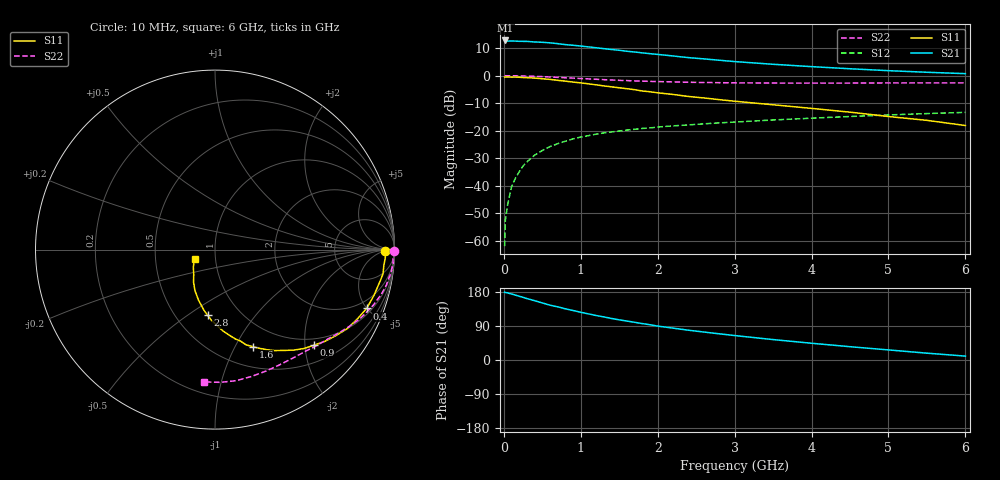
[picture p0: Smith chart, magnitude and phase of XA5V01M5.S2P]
! SIEMENS Discrete & RF Semiconductors
! BFY180
! Si NPN RF Bipolar Junction Transistor in MICRO-X
! VCE = 5 V  IC = 1.5 mA
! Common Emitter S-Parameters:  May  1997
# GHz  S  MA  R  50
!  f  S11  S21  S12  S22
! GHz  MAG  ANG  MAG  ANG  MAG  ANG  MAG  ANG
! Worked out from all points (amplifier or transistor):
!   36 points, 10 MHz to 6 GHz, reference 50 ohm
!   highest |S21| = 12.8 dB at 20 MHz (marker M1)
!   |S21| within 3 dB of that: start of sweep to 1.308 GHz
!   unconditionally stable (mu >= 1): 3.398 GHz to end of sweep
!   at 250 MHz: K = 0.10, MSG = 22.6 dB, |S12| = -32.8 dB
!   at 1.4 GHz: K = 0.58, MSG = 15.0 dB, |S12| = -20.4 dB
!   at 6 GHz: K = 1.06, MAG = 5.5 dB, |S12| = -13.3 dB
!   S11 on the Smith chart (normalised r, x): 10 MHz: 35, -4; 400 MHz: 1.36, -4.99; 900 MHz: 0.85, -2.20; 1.6 GHz: 0.72, -1.18; 2.8 GHz: 0.71, -0.60; 6 GHz: 0.79, -0.08
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0.01  0.9451 -0.4  4.292 179.0  0.0008 78.9  0.9969 -0.3
0.02  0.9477 -1.4  4.372 178.2  0.0024 87.1  0.9999 -0.6
0.05  0.9501 -2.7  4.251 177.0  0.0046 88.2  0.9971 -1.5
0.1  0.9448 -5.4  4.285 174.2  0.0096 87.2  0.9925 -3.0
0.15  0.9457 -8.2  4.252 171.3  0.0137 85.4  0.9958 -4.5
0.25  0.9275 -13.6  4.21 165.4  0.0229 81.2  0.9896 -7.5
0.3  0.9212 -16.2  4.209 162.1  0.0272 79.3  0.983 -8.9
0.4  0.9062 -21.2  4.101 156.5  0.036 76.0  0.9746 -11.7
0.5  0.8806 -26.3  4.05 150.6  0.0438 72.7  0.9626 -14.4
0.6  0.8575 -31.0  3.956 144.7  0.0515 69.7  0.9481 -16.9
0.9  0.7667 -44.0  3.574 130.6  0.0712 61.1  0.9047 -23.9
1.1  0.7122 -51.8  3.338 121.7  0.0815 56.9  0.8752 -27.9
1.4  0.6282 -62.6  2.998 109.6  0.0951 51.4  0.8364 -33.3
1.6  0.5806 -68.7  2.782 102.8  0.1029 48.5  0.8155 -36.4
2  0.4892 -79.8  2.44 89.5  0.1168 43.6  0.7831 -42.2
2.2  0.4569 -84.2  2.284 84.1  0.1227 41.3  0.772 -45.0
2.4  0.4198 -89.0  2.131 78.6  0.1278 39.6  0.7605 -47.6
2.8  0.3675 -96.5  1.911 69.1  0.1392 36.5  0.7474 -52.6
3.5  0.2966 -108.0  1.614 53.9  0.157 31.2  0.7358 -61.2
4.5  0.2177 -123.3  1.338 35.1  0.1816 24.0  0.7356 -74.0
5.5  0.1546 -141.4  1.155 18.0  0.2053 16.5  0.7403 -87.7
6  0.1245 -156.0  1.091 10.3  0.216 12.4  0.7394 -94.7
